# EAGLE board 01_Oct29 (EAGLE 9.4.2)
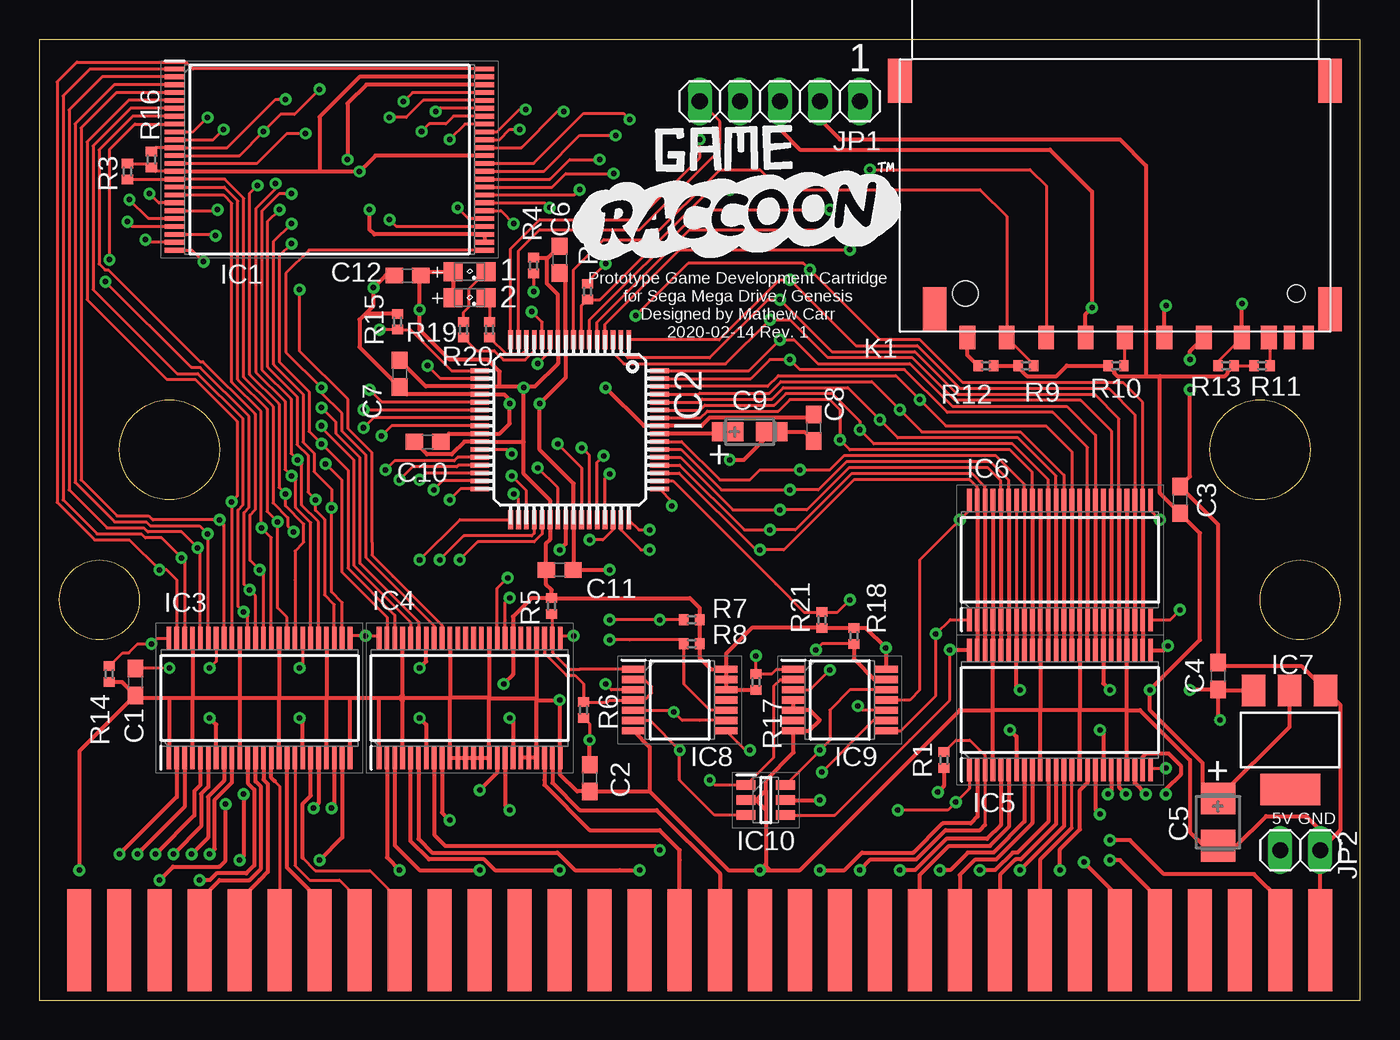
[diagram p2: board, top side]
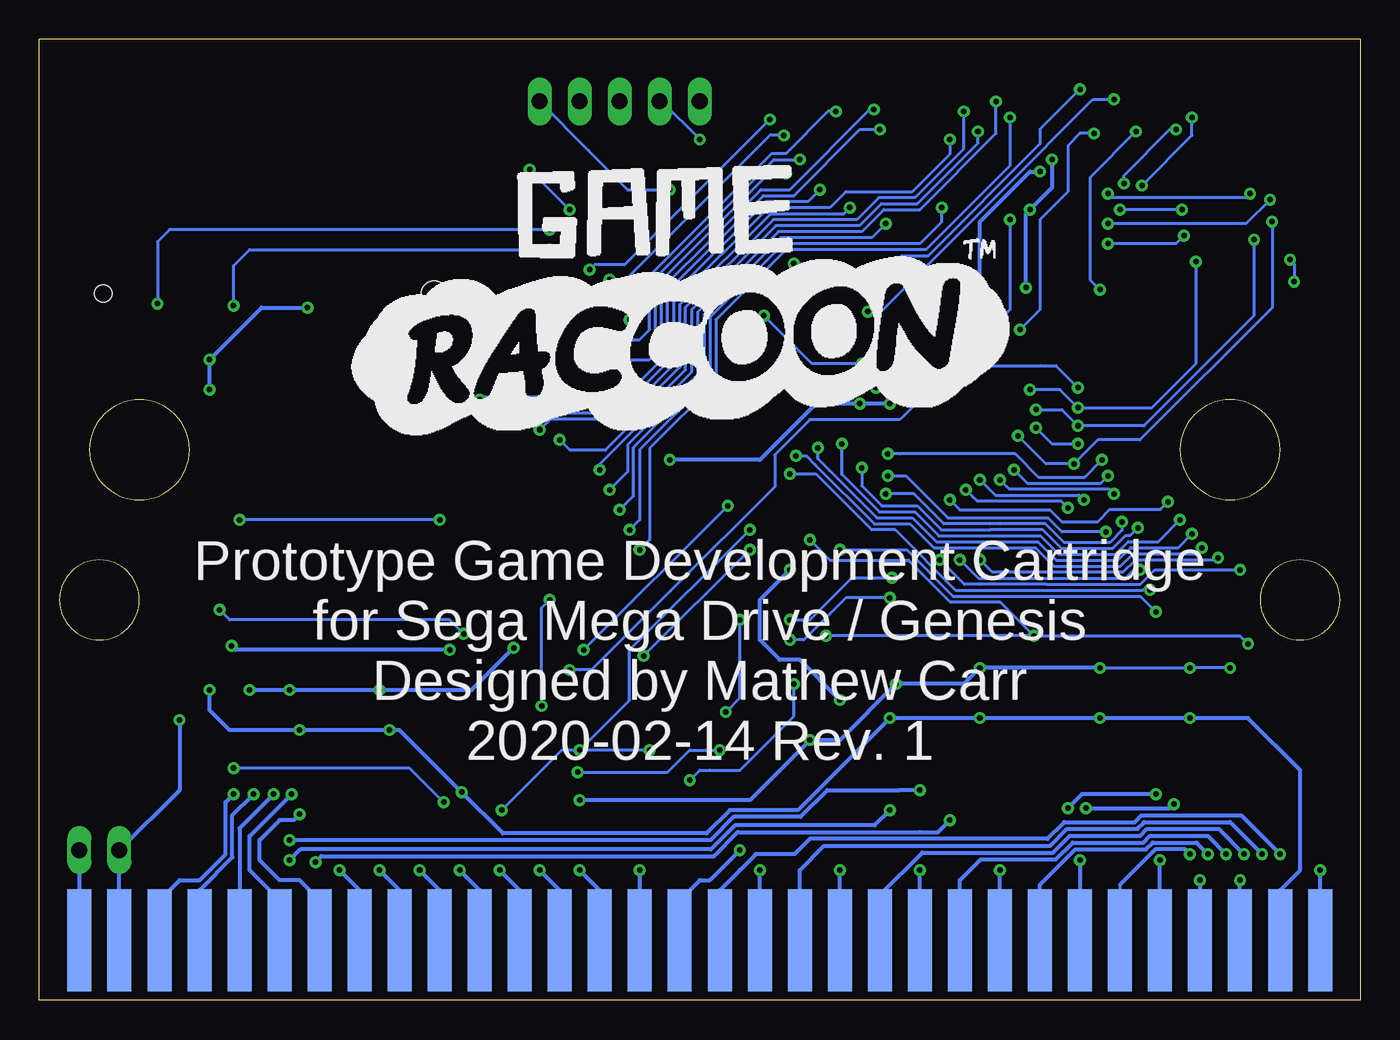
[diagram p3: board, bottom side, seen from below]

Size 83.82 x 60.96 mm. Coordinates in mm from the lower left corner, seen from the top.
Copper layers (1*16): Top 0.035mm / dielectric 1.5mm / Bottom 0.035mm
Design rules "default": minimum track width 6mil, minimum drill 0.35mm, track to track 6mil, track to pad 6mil, pad to pad 6mil, via to via 6mil, smd to smd 6mil, copper to edge 40mil, drill to drill 6mil, minimum pad ring 10mil, minimum via ring 8mil, stop-mask expansion 4mil, vias tented up to drill 0mil, thermal gap 10mil
Net classes: 0 default: width 0.178 mm, clearance 0.178 mm; 1 pow: width 0.254 mm, clearance 0.178 mm

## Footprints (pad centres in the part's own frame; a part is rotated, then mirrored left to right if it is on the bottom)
C0603 = smd 1.1 x 1: 1 -0.85,0; 2 0.85,0
CT3528 = smd 2 x 2.2: + -1.5,0; - 1.5,0
CT3216 = smd 2 x 1.2: + -1.4,0; - 1.4,0
GENESIS-LARGE = smd 1.524 x 6.477 bottom: A1 2.54,3.81; A2 5.08,3.81; A3 7.62,3.81; A4 10.16,3.81; A5 12.7,3.81; A6 15.24,3.81; A7 17.78,3.81; A8 20.32,3.81; A9 22.86,3.81; A10 25.4,3.81; A11 27.94,3.81; A12 30.48,3.81; A13 33.02,3.81; A14 35.56,3.81; A15 38.1,3.81; A16 40.64,3.81; A17 43.18,3.81; A18 45.72,3.81; A19 48.26,3.81; A20 50.8,3.81; A21 53.34,3.81; A22 55.88,3.81; A23 58.42,3.81; A24 60.96,3.81; A25 63.5,3.81; A26 66.04,3.81; A27 68.58,3.81; A28 71.12,3.81; A29 73.66,3.81; A30 76.2,3.81; A31 78.74,3.81; A32 81.28,3.81 | smd 1.524 x 6.477: B1 2.54,3.81; B2 5.08,3.81; B3 7.62,3.81; B4 10.16,3.81; B5 12.7,3.81; B6 15.24,3.81; B7 17.78,3.81; B8 20.32,3.81; B9 22.86,3.81; B10 25.4,3.81; B11 27.94,3.81; B12 30.48,3.81; B13 33.02,3.81; B14 35.56,3.81; B15 38.1,3.81; B16 40.64,3.81; B17 43.18,3.81; B18 45.72,3.81; B19 48.26,3.81; B20 50.8,3.81; B21 53.34,3.81; B22 55.88,3.81; B23 58.42,3.81; B24 60.96,3.81; B25 63.5,3.81; B26 66.04,3.81; B27 68.58,3.81; B28 71.12,3.81; B29 73.66,3.81; B30 76.2,3.81; B31 78.74,3.81; B32 81.28,3.81
SOP50P2000X120-48N = smd 1.25 x 0.3: 1 -9.825,5.75; 2 -9.825,5.25; 3 -9.825,4.75; 4 -9.825,4.25; 5 -9.825,3.75; 6 -9.825,3.25; 7 -9.825,2.75; 8 -9.825,2.25; 9 -9.825,1.75; 10 -9.825,1.25; 11 -9.825,0.75; 12 -9.825,0.25; 13 -9.825,-0.25; 14 -9.825,-0.75; 15 -9.825,-1.25; 16 -9.825,-1.75; 17 -9.825,-2.25; 18 -9.825,-2.75; 19 -9.825,-3.25; 20 -9.825,-3.75; 21 -9.825,-4.25; 22 -9.825,-4.75; 23 -9.825,-5.25; 24 -9.825,-5.75; 25 9.825,-5.75; 26 9.825,-5.25; 27 9.825,-4.75; 28 9.825,-4.25; 29 9.825,-3.75; 30 9.825,-3.25; 31 9.825,-2.75; 32 9.825,-2.25; 33 9.825,-1.75; 34 9.825,-1.25; 35 9.825,-0.75; 36 9.825,-0.25; 37 9.825,0.25; 38 9.825,0.75; 39 9.825,1.25; 40 9.825,1.75; 41 9.825,2.25; 42 9.825,2.75; 43 9.825,3.25; 44 9.825,3.75; 45 9.825,4.25; 46 9.825,4.75; 47 9.825,5.25; 48 9.825,5.75
TQFP64-10X10 = smd 1.2 x 0.3: 1 -5.7,3.75; 2 -5.7,3.25; 3 -5.7,2.75; 4 -5.7,2.25; 5 -5.7,1.75; 6 -5.7,1.25; 7 -5.7,0.75; 8 -5.7,0.25; 9 -5.7,-0.25; 10 -5.7,-0.75; 11 -5.7,-1.25; 12 -5.7,-1.75; 13 -5.7,-2.25; 14 -5.7,-2.75; 15 -5.7,-3.25; 16 -5.7,-3.75; 33 5.7,-3.75; 34 5.7,-3.25; 35 5.7,-2.75; 36 5.7,-2.25; 37 5.7,-1.75; 38 5.7,-1.25; 39 5.7,-0.75; 40 5.7,-0.25; 41 5.7,0.25; 42 5.7,0.75; 43 5.7,1.25; 44 5.7,1.75; 45 5.7,2.25; 46 5.7,2.75; 47 5.7,3.25; 48 5.7,3.75 | smd 0.3 x 1.2: 17 -3.75,-5.7; 18 -3.25,-5.7; 19 -2.75,-5.7; 20 -2.25,-5.7; 21 -1.75,-5.7; 22 -1.25,-5.7; 23 -0.75,-5.7; 24 -0.25,-5.7; 25 0.25,-5.7; 26 0.75,-5.7; 27 1.25,-5.7; 28 1.75,-5.7; 29 2.25,-5.7; 30 2.75,-5.7; 31 3.25,-5.7; 32 3.75,-5.7; 49 3.75,5.7; 50 3.25,5.7; 51 2.75,5.7; 52 2.25,5.7; 53 1.75,5.7; 54 1.25,5.7; 55 0.75,5.7; 56 0.25,5.7; 57 -0.25,5.7; 58 -0.75,5.7; 59 -1.25,5.7; 60 -1.75,5.7; 61 -2.25,5.7; 62 -2.75,5.7; 63 -3.25,5.7; 64 -3.75,5.7
SOP50P810X120-48N = smd 1.475 x 0.3: 1 -3.788,5.75; 2 -3.788,5.25; 3 -3.788,4.75; 4 -3.788,4.25; 5 -3.788,3.75; 6 -3.788,3.25; 7 -3.788,2.75; 8 -3.788,2.25; 9 -3.788,1.75; 10 -3.788,1.25; 11 -3.788,0.75; 12 -3.788,0.25; 13 -3.788,-0.25; 14 -3.788,-0.75; 15 -3.788,-1.25; 16 -3.788,-1.75; 17 -3.788,-2.25; 18 -3.788,-2.75; 19 -3.788,-3.25; 20 -3.788,-3.75; 21 -3.788,-4.25; 22 -3.788,-4.75; 23 -3.788,-5.25; 24 -3.788,-5.75; 25 3.788,-5.75; 26 3.788,-5.25; 27 3.788,-4.75; 28 3.788,-4.25; 29 3.788,-3.75; 30 3.788,-3.25; 31 3.788,-2.75; 32 3.788,-2.25; 33 3.788,-1.75; 34 3.788,-1.25; 35 3.788,-0.75; 36 3.788,-0.25; 37 3.788,0.25; 38 3.788,0.75; 39 3.788,1.25; 40 3.788,1.75; 41 3.788,2.25; 42 3.788,2.75; 43 3.788,3.25; 44 3.788,3.75; 45 3.788,4.25; 46 3.788,4.75; 47 3.788,5.25; 48 3.788,5.75
SOT223 = smd 1.499 x 2.007: 1 -2.261,-3.15; 2 0.025,-3.15; 3 2.311,-3.15 | smd 3.81 x 2.007: 4 0,3.15
SOP65P640X120-14N = smd 1.475 x 0.45: 1 -2.938,1.95; 2 -2.938,1.3; 3 -2.938,0.65; 4 -2.938,0; 5 -2.938,-0.65; 6 -2.938,-1.3; 7 -2.938,-1.95; 8 2.938,-1.95; 9 2.938,-1.3; 10 2.938,-0.65; 11 2.938,0; 12 2.938,0.65; 13 2.938,1.3; 14 2.938,1.95
SOT95P280X145-6N = smd 1.2 x 0.6: 1 -1.25,0.95; 2 -1.25,0; 3 -1.25,-0.95; 4 1.25,-0.95; 5 1.25,0; 6 1.25,0.95
1X05 = drill 1.016 long: 1 -5.08,0; 2 -2.54,0; 3 0,0; 4 2.54,0; 5 5.08,0
1X02 = drill 1.016 long: 1 -1.27,0; 2 1.27,0
693063020911 = smd 1 x 1.5: 1 19.125,0; 2 16.625,0; 3 14.125,0; 4 11.625,0; 5 9.125,0; 6 6.625,0; 7 4.2,0; 8 2.5,0; 9 21.625,0 | smd 0.7 x 1.5: CD 1.2,0; WP 0,0 | smd 1.5 x 2.8: P$12 -1.4,-1.8; P$13 23.7,-1.8; P$14 -1.4,-16.3; P$15 25.9,-16.3 | hole 1.1: 0.75,-2.8 | hole 1.6: 21.75,-2.8
SML0805 = smd 1.2 x 1.2: A 1.05,0; C -1.05,0
R0402 = smd 0.6 x 0.7: 1 -0.5,0; 2 0.5,0

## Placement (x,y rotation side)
C1  100nF  [C0603]  6.1,20.19 270 top
C2  100nF  [C0603]  34.92,14.1 270 top
C3  100nF  [C0603]  72.39,31.75 90 top
C4  100nF  [C0603]  74.8,20.57 270 top
C5  22uF_16V_Tantalum  [CT3528]  74.8,11.3 270 top
C6  100nF  [C0603]  33.02,46.99 270 top
C7  100nF  [C0603]  22.86,39.75 270 top
C8  100nF  [C0603]  49.15,36.32 90 top
C9  10uF_10V_Tantalum  [CT3216]  45.09,36.07 0 top
C10  100nF  [C0603]  24.64,35.43 180 top
C11  100nF  [C0603]  33.02,27.3 0 top
C12  100nF  [C0603]  23.37,45.97 180 top
EDGE1  GENESIS-LARGE  [GENESIS-LARGE]  0,0 0 top
IC1  S29GL064S70TFI030  [SOP50P2000X120-48N]  18.41,53.34 0 top
IC2  PIC24FJ64GA006  [TQFP64-10X10]  33.66,36.2 270 top
IC3  SN74ALVC164245DGGR  [SOP50P810X120-48N]  13.97,19.18 90 top
IC4  SN74ALVC164245DGGR  [SOP50P810X120-48N]  27.3,19.18 90 top
IC5  SN74ALVC164245DGGR  [SOP50P810X120-48N]  64.77,18.41 90 top
IC6  74LVC16374ADGG  [SOP50P810X120-48N]  64.77,27.94 90 top
IC7  REG1117  [SOT223]  79.38,16.51 180 top
IC8  SN74LVC32APW  [SOP65P640X120-14N]  40.64,19.05 0 top
IC9  SN74LVC08APWT  [SOP65P640X120-14N]  50.8,19.05 0 top
IC10  SN74LVC1G11DBVR  [SOT95P280X145-6N]  46.1,12.7 0 top
JP1  [1X05]  46.99,57.02 180 top
JP2  [1X02]  80.01,9.53 0 top
K1  693063020911  [693063020911]  80.52,42.04 180 top
LED1  150080BS75000_BLUE  [SML0805]  27.3,46.23 180 top
LED2  MCL-S270GC_GREEN  [SML0805]  27.3,44.58 180 top
R1  10k  [R0402]  57.4,15.24 90 top
R2  2.2k  [R0402]  34.8,44.96 270 top
R3  10k  [R0402]  5.59,52.58 90 top
R4  10k  [R0402]  31.37,46.61 90 top
R5  10k  [R0402]  32.51,25.02 90 top
R6  10k  [R0402]  34.54,18.41 270 top
R7  10k  [R0402]  41.4,24.13 0 top
R8  10k  [R0402]  41.4,22.61 0 top
R9  10k  [R0402]  62.61,40.26 180 top
R10  10R  [R0402]  68.33,40.26 0 top
R11  10k  [R0402]  77.6,40.26 0 top
R12  10k  [R0402]  60.07,40.26 180 top
R13  10k  [R0402]  75.31,40.26 0 top
R14  10k  [R0402]  4.45,20.7 270 top
R15  10k  [R0402]  22.73,43.05 90 top
R16  10k  [R0402]  7.11,53.34 270 top
R17  10k  [R0402]  45.47,20.19 270 top
R18  10k  [R0402]  51.69,23.11 90 top
R19  330R  [R0402]  26.92,42.55 270 top
R20  150R  [R0402]  28.57,42.55 270 top
R21  10k  [R0402]  49.66,24.13 270 top
U$1  [GAMERACCOONLOGO3_800DPI]  33.15,46.48 0 top
U$2  [GAMERACCOONLOGO2_REVERSEBACK_400DPI]  20.95,34.92 0 top

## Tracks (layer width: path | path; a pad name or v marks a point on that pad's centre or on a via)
CART_!C_CE
  Top 0.203: R5.1 32.55,24.48 IC4.26 32.55,22.05 33.61,21 34.29,21 IC8.1
CART_!C_OE
  Top 0.203: IC8.2 38.41,20.35 38.86,19.9 38.86,19.5 38.41,19.05 IC8.4 36.2,19.05 36.06,18.91 R6.1 34.54,20.07 33.99,20.62 33.45,20.62 32.05,22.02 IC4.27
CART_!LDS  (via drill 0.35)
  Top 0.203: IC8.10 42.56,18.4 40.9,20.06 R8.1 40.65,22.86 37.47,22.86 v36.2,22.86 | IC4.32 29.55,24.13 29.55,25.24 v29.84,25.53
  Bottom 0.203: v29.84,25.53 32.64,25.53 35.31,22.86 v36.2,22.86
CART_!TIME  (via drill 0.35)
  Top 0.203: R7.1 v39.37,24.13 v36.2,24.13 | IC8.9 41.91,17.75 40.8,17.75 v40.26,18.29 40.15,18.4 IC8.5 | IC4.33 29.05,26.13 v29.72,26.8
  Bottom 0.203: v40.26,18.29 39.37,19.18 v39.37,24.13 | v36.2,24.13 34.92,24.13 32.26,26.8 v29.72,26.8
CART_!VRES  (via drill 0.35)
  Top 0.203: R2.1 34.8,45.59 v35.94,46.74 | R4.1 v31.37,44.96 | v17.78,57.78 16.19,56.2 15.3,56.2 v14.22,55.12 12.7,53.59 IC1.12 | v16.51,45.09 16.51,43.18 16.51,41.19 19.58,38.12 19.58,36.27 21.11,34.74 21.11,29.21 21.11,29.06 21.11,28.24 22.45,26.89 25.55,23.79 IC4.40
  Bottom 0.203: v35.94,46.74 33.15,46.74 v31.37,44.96 29.08,47.24 27.4,47.24 20.32,54.33 20.32,55.24 v17.78,57.78 | v14.22,55.12 17.14,52.2 17.14,45.72 v16.51,45.09
CART_A0  (via drill 0.35)
  Top 0.203: IC1.25 17.11,47.59 15.64,46.12 15.64,41.12 v17.91,38.86 17.91,38.52 19.2,37.23 19.2,36.11 20.72,34.58 20.72,28.08 25.05,23.75 IC4.41 | IC2.18 25.45,39.45 v24.64,40.26
  Bottom 0.203: v24.64,40.26 20.32,40.26 19.3,40.26 v17.91,38.86
CART_A1  (via drill 0.35)
  Top 0.203: IC1.24 9.69,47.59 v10.41,46.86 | IC4.43 24.05,24.01 20.34,27.73 20.34,34.42 18.82,35.95 18.82,36.68 v17.91,37.59 | IC2.21 21.75,37.95 v20.95,38.73
  Bottom 0.203: v10.41,46.86 10.41,40.39 13.21,37.59 v17.91,37.59 19.05,38.73 v20.95,38.73
CART_A2  (via drill 0.35)
  Top 0.203: IC1.23 6.9,48.09 v6.73,48.26 | IC4.44 23.55,23.97 19.96,27.57 19.96,34.27 17.91,36.32 v17.91,36.45 | IC2.22 20.59,37.45 v20.57,37.47
  Bottom 0.203: v6.73,48.26 6.73,43.43 13.72,36.45 v17.91,36.45 18.92,37.47 v20.57,37.47
CART_A3  (via drill 0.35)
  Top 0.203: IC1.22 11.1,48.59 v11.18,48.51 | IC4.46 22.55,24.43 19.58,27.41 19.58,33.63 v17.91,35.31 17.12,36.09 17.12,38.62 15.26,40.48 15.26,47.27 v16,48.01 | IC2.23 21.2,36.95 v20.57,36.32
  Bottom 0.203: v11.18,48.51 11.68,48.01 v16,48.01 | v20.57,36.32 19.56,35.31 v17.91,35.31
CART_A4  (via drill 0.35)
  Top 0.203: IC1.21 5.9,49.09 v5.59,49.4 | IC4.47 22.05,24.3 19.2,27.16 19.2,33 v18.16,34.04 | IC2.24 22.35,36.45 v21.72,35.81
  Bottom 0.203: v5.59,49.4 5.59,43.94 13.97,35.56 16.64,35.56 v18.16,34.04 19.94,34.04 v21.72,35.81
CART_A5  (via drill 0.35)
  Top 0.203: IC3.26 19.22,25.23 18.54,25.91 v18.54,31.24 18.54,32.43 17.42,33.55 17.42,34.72 16.74,35.4 16.74,38.46 14.88,40.32 14.88,48.16 v16,49.28 | IC1.20 6.92,49.59 v5.71,50.8 | IC2.31 25.58,32.95 v25.02,32.38
  Bottom 0.203: v5.71,50.8 7.24,49.28 v16,49.28 | v18.54,31.24 18.97,31.67 24.3,31.67 24.57,31.94 v25.02,32.38
CART_A6  (via drill 0.35)
  Top 0.203: IC1.19 11.23,50.09 v11.3,50.16 | v15.24,50.16 14.5,49.43 14.5,40.16 16.36,38.3 16.36,35.24 17.04,34.56 17.04,32.23 v17.53,31.75 17.53,31.08 18.1,30.5 18.1,25.71 18.72,25.09 IC3.27 | IC2.30 24.55,33.45 v24.13,33.02
  Bottom 0.203: v11.3,50.16 v15.24,50.16 | v24.13,33.02 23.16,32.05 17.82,32.05 v17.53,31.75
CART_A7  (via drill 0.35)
  Top 0.203: v16,51.18 15.23,51.18 14.12,50.07 14.12,40 15.98,38.15 15.98,34.7 v16.38,34.29 16.66,34.01 16.66,31.41 17.72,30.35 IC3.29 | IC1.18 7.58,50.59 v6.99,51.18 | IC2.27 29.7,34.95 v29.97,34.67
  Bottom 0.203: v6.99,51.18 7.24,50.93 15.75,50.93 v16,51.18 | v29.97,34.67 29.21,34.67 21.89,34.67 20.4,33.19 17.48,33.19 v16.38,34.29
CART_A8  (via drill 0.35)
  Top 0.203: v4.45,46.99 4.45,53.98 6.06,55.59 IC1.8 | IC3.37 13.72,25.65 v13.34,26.04 12.98,26.39 12.98,30.94 13.31,31.27 13.31,37.04 10.22,40.13 9.65,40.13 v4.19,45.59 | IC2.45 35.91,33.11 v36.2,33.4
  Bottom 0.203: v4.45,46.99 4.19,46.74 v4.19,45.59 | v13.34,26.04 13.77,26.04 13.79,26.01 25.67,26.01 29.5,29.84 30.98,29.84 34.54,33.4 v36.2,33.4
CART_A9  (via drill 0.35)
  Top 0.203: IC3.36 14.22,27.05 v13.97,27.3 13.36,27.91 13.36,30.79 13.69,31.11 13.69,37.2 10.38,40.51 10.2,40.51 4.38,46.33 4.17,46.33 3.79,46.72 3.79,53.95 5.92,56.09 IC1.7 | IC2.36 31.41,29.63 31.24,29.46 26.92,29.46 v25.4,27.94
  Bottom 0.203: v13.97,27.3 14.36,27.3 14.89,26.77 23.5,26.77 24.23,26.77 v25.4,27.94
CART_A10  (via drill 0.35)
  Top 0.203: IC3.38 13.22,24.37 v12.95,24.64 12.6,24.99 12.6,31.1 12.93,31.43 12.93,36.88 10.06,39.75 8.74,39.75 3.4,45.09 3.4,54.2 5.79,56.59 IC1.6
  Top 0.254: v33.02,28.57 33.41,28.96 IC2.40
  Bottom 0.203: v12.95,24.64 13.95,25.63 25.83,25.63 28.77,28.57 v33.02,28.57
CART_A11  (via drill 0.35)
  Top 0.203: IC3.40 12.22,31.59 v12.19,31.62 12.55,31.98 12.55,36.73 9.9,39.37 8.1,39.37 3.02,44.45 3.02,54.46 5.66,57.09 IC1.5 | IC2.32 26.73,32.45 v26.04,31.75
  Bottom 0.203: v12.19,31.62 12.68,31.14 15.88,31.14 16.66,30.35 18.92,30.35 19.68,31.11 25.4,31.11 v26.04,31.75
CART_A12  (via drill 0.35)
  Top 0.203: IC3.41 11.72,30.19 v11.43,30.48 7.19,30.48 6.94,30.73 4.93,30.73 2.64,33.02 2.64,55.35 4.88,57.59 IC1.4 | v32.89,35.31 34.41,33.79 IC2.42
  Bottom 0.203: v11.43,30.48 12.8,29.11 14.72,29.11 15.52,28.3 19.12,28.3 20.29,29.46 26.73,29.46 28.26,30.99 30.51,30.99 32.89,33.37 v32.89,35.31
CART_A13  (via drill 0.35)
  Top 0.203: IC3.43 10.72,29.54 v10.67,29.59 10.16,30.1 7.03,30.1 6.78,30.35 4.77,30.35 2.26,32.86 2.26,55.6 4.75,58.09 IC1.3 | v34.42,35.05 34.91,34.56 IC2.43
  Bottom 0.203: v10.67,29.59 11.53,28.73 14.56,28.73 15.37,27.92 19.28,27.92 20.13,28.77 20.19,28.83 20.44,29.08 24.13,29.08 26.89,29.08 28.41,30.61 30.67,30.61 33.69,33.62 34.42,34.35 v34.42,35.05
CART_A14  (via drill 0.35)
  Top 0.203: IC3.44 10.22,28.52 v10.03,28.7 9.02,29.72 6.88,29.72 6.62,29.97 4.29,29.97 1.88,32.38 1.88,56.49 3.98,58.59 IC1.2 | IC2.44 35.41,34.13 v35.81,34.54
  Bottom 0.203: v10.03,28.7 10.39,28.34 14.4,28.34 15.21,27.54 19.43,27.54 20.6,28.7 23.5,28.7 27.05,28.7 28.57,30.23 30.83,30.23 34.59,33.99 35.14,34.54 v35.81,34.54
CART_A15  (via drill 0.35)
  Top 0.203: IC3.46 9.22,27.86 v9.02,28.07 7.75,29.34 6.72,29.34 6.46,29.59 3.66,29.59 1.5,31.75 1.5,57.38 3.21,59.09 IC1.1 | v24.13,27.94 26.68,30.5 IC2.33
  Bottom 0.203: v9.02,28.07 9.12,27.96 14.24,27.96 15.05,27.16 23.34,27.16 v24.13,27.94
CART_A16  (via drill 0.35)
  Top 0.203: IC3.47 8.72,26.67 8.09,27.3 v7.62,27.3 5.71,29.21 3.5,29.21 1.12,31.59 1.12,58.27 2.37,59.52 9.33,59.52 9.76,59.09 IC1.48 | IC2.37 31.91,29.59 31.4,29.08 27.81,29.08 v26.67,27.94
  Bottom 0.203: v7.62,27.3 13.04,27.3 13.95,26.39 19.68,26.39 19.91,26.39 24.13,26.39 25.12,26.39 v26.67,27.94
CART_A17  (via drill 0.35)
  Top 0.203: IC3.35 14.72,29.35 v14.1,29.97 14.07,30 14.07,37.36 12.21,39.22 12.21,50.56 11.69,51.09 IC1.17 | IC2.39 32.91,32.5 v31.62,33.78
  Bottom 0.203: v14.1,29.97 14.58,29.49 14.87,29.49 15.68,28.68 18.96,28.68 20.13,29.84 23.5,29.84 26.57,29.84 28.1,31.37 30.35,31.37 31.62,32.64 v31.62,33.78
CART_A18  (via drill 0.35)
  Top 0.203: IC1.16 11.73,51.59 12.6,50.72 12.6,39.37 14.45,37.52 14.45,31.01 v15.11,30.35 15.11,27.94 15.11,24.89 15.72,24.29 IC3.33 | IC2.34 30.41,31.82 v30.1,32.13
  Bottom 0.203: v15.11,30.35 15.11,29.8 15.86,29.06 18.8,29.06 19.97,30.23 22.86,30.23 23.5,30.23 26.42,30.23 28.32,32.13 v30.1,32.13
CART_A19  (via drill 0.35)
  Top 0.203: IC1.9 9.75,55.09 v10.67,56.01 | IC3.32 16.22,26.67 16.22,28.5 16.79,29.07 16.79,30.2 15.62,31.37 v15.62,32.13 15.21,32.54 15.21,37.83 13.36,39.69 13.36,51.2 v13.84,51.69 | IC2.29 26.59,33.95 26.49,33.84 23.68,33.84 v22.86,33.02
  Bottom 0.203: v13.84,51.69 10.67,54.86 v10.67,56.01 | v15.62,32.13 15.92,32.43 22.27,32.43 v22.86,33.02
CART_A20  (via drill 0.35)
  Top 0.203: v14.99,51.82 14.99,51.48 13.74,50.23 13.74,39.85 15.6,37.99 15.6,33.68 v16,33.27 16.28,33 16.28,31.25 17.22,30.31 IC3.30 | IC1.10 11.03,54.59 v11.68,55.24 | IC2.28 26.56,34.45 26.33,34.22 22.54,34.22 v21.97,33.66
  Bottom 0.203: v14.99,51.82 14.99,52.32 12.06,55.24 v11.68,55.24 | v21.97,33.66 21.12,32.81 16.47,32.81 v16,33.27
CART_D0  (via drill 0.35)
  Top 0.203: IC2.52 40.64,33.95 44.74,29.84 v46.35,29.84 47.97,29.84 51.53,33.4 59.21,33.4 60.02,32.59 IC6.46 | v26.54,50.29 27.25,49.59 IC1.29
  Top 0.254: IC6.46 IC6.3 IC5.46
  Bottom 0.203: v46.35,29.84 45.72,30.48 45.72,34.92 41.27,39.37 41.27,43.34 36.61,48.01 27.94,48.01 26.54,49.4 v26.54,50.29
CART_D1  (via drill 0.35)
  Top 0.203: IC2.59 41.92,37.45 42.23,37.76 46.65,37.76 47.37,38.48 50.32,38.48 52.07,36.73 v52.07,36.2 52.96,35.31 61.75,35.31 64.02,33.04 IC6.38 | v32.38,50.29 32.09,50.59 IC1.31
  Top 0.254: IC6.38 IC6.11 IC5.38
  Bottom 0.203: v52.07,36.2 51.36,36.91 46.43,36.91 43.18,40.16 43.18,44.13 37.4,49.91 32.77,49.91 v32.38,50.29
CART_D2  (via drill 0.35)
  Top 0.203: IC6.32 67.02,35.85 65.2,37.67 57.96,37.67 55.25,40.39 49.4,40.39 47.88,41.91 v46.99,41.91 45.02,39.95 IC2.64 | v36.45,52.45 33.4,52.45 32.54,51.59 IC1.33
  Top 0.254: IC6.32 IC6.17 IC5.32
  Bottom 0.203: v46.99,41.91 45.72,41.91 45.09,42.55 45.09,44.92 37.55,52.45 v36.45,52.45
CART_D3  (via drill 0.35)
  Top 0.203: IC6.27 69.52,37.16 67.86,38.82 58.43,38.82 55.72,41.53 51.82,41.53 v47.62,45.72 46.96,45.72 43.13,41.9 IC2.1 | v36.58,54.86 34.29,54.86 32.02,52.59 IC1.35
  Top 0.254: IC6.27 IC6.22 IC5.27
  Bottom 0.203: v47.62,45.72 46.61,45.72 37.47,54.86 v36.58,54.86
CART_D4  (via drill 0.35)
  Top 0.203: IC6.29 68.52,36.89 66.97,38.44 58.28,38.44 55.56,41.15 50.29,41.15 v46.99,44.45 46.23,44.45 42.53,40.76 37.35,40.76 36.91,41.2 IC2.2 | v33.27,56.39 32.89,56.39 30.59,54.09 IC1.38
  Top 0.254: IC6.29 IC6.20 IC5.29
  Bottom 0.203: v46.99,44.45 46.63,44.45 37.36,53.72 36.45,53.72 33.78,56.39 v33.27,56.39
CART_D5  (via drill 0.35)
  Top 0.203: IC6.33 66.52,35.08 64.31,37.29 57.62,37.29 54.91,40.01 48.26,40.01 v47.62,40.64 46.35,40.64 45.16,39.45 IC2.63 | v30.86,56.52 30.48,56.52 29.05,55.09 IC1.40
  Top 0.254: IC6.33 IC6.16 IC5.33
  Bottom 0.203: v47.62,40.64 45.09,40.64 44.7,41.02 44.7,44.76 40.6,48.86 38.03,51.44 36.2,51.44 31.11,56.52 v30.86,56.52
CART_D6  (via drill 0.35)
  Top 0.203: IC6.8 IC6.41 62.52,32.73 60.71,34.54 51.05,34.54 50.16,33.66 v48.26,33.66 45.72,33.66 45.09,33.02 43.18,33.02 40.76,35.45 IC2.55 | v24.26,55.12 24.74,55.6 25.8,55.6 26.29,56.09 IC1.42
  Top 0.254: IC6.8 IC5.41
  Bottom 0.203: v48.26,33.66 48.26,34 42.42,39.84 42.42,43.81 37.08,49.15 31.78,49.15 30.38,50.55 28.1,50.55 24.26,54.39 v24.26,55.12
CART_D7  (via drill 0.35)
  Top 0.203: IC2.51 40.6,33.45 45.47,28.57 v45.72,28.57 47.24,28.57 51.69,33.02 59.05,33.02 59.52,32.55 IC6.47 | v22.23,56.01 23.28,56.01 24.36,57.09 IC1.44
  Top 0.254: IC6.47 IC6.2 IC5.47
  Bottom 0.203: v45.72,28.57 45.09,29.21 45.09,30.48 45.09,35.02 40.89,39.21 40.89,43.18 36.45,47.62 27.56,47.62 22.23,52.96 v22.23,56.01
CART_D8  (via drill 0.35)
  Top 0.203: IC2.53 40.68,34.45 44.01,31.11 v46.99,31.11 48.7,31.11 51.37,33.78 60.2,33.78 61.02,32.96 IC6.44 | v30.1,49.28 29.29,50.09 IC1.30
  Top 0.254: IC6.44 IC6.5 IC5.44
  Bottom 0.203: v46.99,31.11 46.1,32 46.1,35.08 41.66,39.53 41.66,43.5 36.77,48.39 30.99,48.39 v30.1,49.28
CART_D9  (via drill 0.35)
  Top 0.203: IC2.61 41.84,38.45 41.92,38.52 46.34,38.52 47.05,39.24 52.83,39.24 v54.61,37.47 56.01,36.07 62.26,36.07 65.02,33.31 IC6.36 | v34.29,51.44 33.95,51.09 IC1.32
  Top 0.254: IC6.36 IC6.13 IC5.36
  Bottom 0.203: v54.61,37.47 54.41,37.67 46.75,37.67 43.94,40.48 43.94,44.44 37.71,50.67 35.05,50.67 v34.29,51.44
CART_D10  (via drill 0.35)
  Top 0.203: IC6.30 68.02,36.12 66.08,38.05 58.12,38.05 55.41,40.77 50.04,40.77 47.62,43.18 v46.35,43.18 43.55,40.37 37.1,40.37 36.41,41.06 IC2.3 | v35.56,53.34 33.66,53.34 32.41,52.09 IC1.34
  Top 0.254: IC6.30 IC6.19 IC5.30
  Bottom 0.203: v46.35,43.18 45.47,44.07 45.47,45.07 37.2,53.34 v35.56,53.34
CART_D11  (via drill 0.35)
  Top 0.203: IC6.26 70.02,37.93 68.75,39.2 58.59,39.2 55.88,41.91 53.34,41.91 v48.9,46.35 48.49,46.76 41.17,46.76 v37.85,43.43 | IC2.11 32.41,41.17 v31.62,40.39 | v37.47,55.88 37.08,56.26 34.54,56.26 31.37,53.09 IC1.36
  Top 0.254: IC6.26 IC6.23 IC5.26
  Bottom 0.203: v31.62,40.39 34.8,40.39 v37.85,43.43 | v48.9,46.35 48.6,46.65 46.7,46.65 v37.47,55.88
CART_D12  (via drill 0.35)
  Top 0.203: IC6.35 65.52,34.81 63.88,36.45 57.53,36.45 v55.88,38.1 54.36,39.62 46.9,39.62 46.22,38.95 IC2.62 | v30.48,55.24 29.84,55.24 29.19,54.59 IC1.39
  Top 0.254: IC6.35 IC6.14 IC5.35
  Bottom 0.203: v55.88,38.1 55.69,38.29 46.67,38.29 44.32,40.63 44.32,44.6 37.87,51.05 35.94,51.05 31.75,55.24 v30.48,55.24
CART_D13  (via drill 0.35)
  Top 0.203: IC2.60 41.88,37.95 42.08,38.14 46.49,38.14 47.21,38.86 51.31,38.86 v53.34,36.83 54.48,35.69 62.1,35.69 64.52,33.27 IC6.37 | v26.04,54.61 27.02,55.59 IC1.41
  Top 0.254: IC6.37 IC6.12 IC5.37
  Bottom 0.203: v53.34,36.83 52.88,37.29 46.59,37.29 43.56,40.32 43.56,44.28 37.55,50.29 33.66,50.29 32.64,51.31 28.41,51.31 26.04,53.69 v26.04,54.61
CART_D14  (via drill 0.35)
  Top 0.203: IC2.58 41.96,36.95 42.39,37.38 46.9,37.38 47.62,38.1 50.16,38.1 50.8,37.47 v50.8,35.56 51.44,34.92 61.59,34.92 63.02,33.5 IC6.40 | IC1.43 25.35,56.59 v25.15,56.39
  Top 0.254: IC6.40 IC6.9 IC5.40
  Bottom 0.203: v25.15,56.39 25.15,54.04 28.26,50.93 30.54,50.93 31.94,49.53 37.24,49.53 42.8,43.97 42.8,40 47.88,34.92 50.16,34.92 v50.8,35.56
CART_D15  (via drill 0.35)
  Top 0.203: IC2.54 40.72,34.95 43.28,32.38 v47.62,32.38 49.43,32.38 51.21,34.16 60.36,34.16 61.52,33 IC6.43 | v23.11,57.02 23.68,57.59 IC1.45
  Top 0.254: IC6.43 IC6.6 IC5.43
  Bottom 0.203: v47.62,32.38 46.48,33.53 46.48,35.24 42.04,39.69 42.04,43.65 36.92,48.77 31.62,48.77 30.23,50.16 27.94,50.16 23.11,54.99 v23.11,57.02
DATATRANSCEIVER!OE  (via drill 0.35)
  Top 0.203: IC10.4 50.48,11.75 55.24,16.51 57.78,19.05 v57.78,22.23
  Top 0.254: IC5.25 71.35,22.2 v71.63,22.48 | v57.78,22.23 59,22.23 IC5.48
  Bottom 0.254: v57.78,22.23 71.37,22.23 v71.63,22.48
EDGE_!C_CE
  Top 0.254: EDGE1.B17 43.18,8.05 39.17,12.06 34.29,12.06 32.55,13.8 IC4.23
EDGE_!C_OE
  Top 0.254: EDGE1.B16 40.64,8.89 40.64,9.53 39.37,10.79 34.92,10.79 32.05,13.66 32.05,13.97 IC4.22
EDGE_!LDS  (via drill 0.35)
  Top 0.254: EDGE1.B28 71.12,6.35 68.58,8.89 v67.94,8.89 | IC4.17 29.55,12.36 v29.84,12.06
  Bottom 0.254: v67.94,8.89 67.26,9.58 41.2,9.58 39.68,11.1 30.81,11.1 v29.84,12.06
EDGE_!TIME  (via drill 0.35)
  Top 0.254: EDGE1.B31 78.74,6.35 77.09,8 71.37,8 69.22,10.16 v67.94,10.16 | IC4.16 29.05,14.45 v27.94,13.34
  Bottom 0.254: v67.94,10.16 41.23,10.16 39.75,11.63 35.51,11.63 33.81,13.34 29.21,13.34 v27.94,13.34
EDGE_!VRES  (via drill 0.35)
  Top 0.254: EDGE1.B27 68.58,6.48 v66.29,8.76 | IC4.9 25.55,11.91 v26.04,11.43
  Bottom 0.254: v66.29,8.76 65.91,9.14 41.02,9.14 39.5,10.66 27.94,10.66 26.8,10.66 v26.04,11.43
EDGE_A1  (via drill 0.35)
  Top 0.254: IC4.8 25.05,10.51 25.76,9.8 39.09,9.8 v39.37,9.53
  Bottom 0.254: v39.37,9.53 41.27,7.62 41.91,7.62 43.18,6.35 EDGE1.A17
EDGE_A2  (via drill 0.35)
  Top 0.254: v38.1,8.26 36.83,8.26 33.99,8.26 32.87,9.37 24.92,9.37 24.05,10.23 IC4.6
  Bottom 0.254: EDGE1.A15 v38.1,8.26
EDGE_A3  (via drill 0.35)
  Top 0.254: v33.02,8.26 28.91,8.26 28.22,8.94 24.72,8.94 23.55,10.1 IC4.5
  Bottom 0.254: EDGE1.A13 v33.02,8.26
EDGE_A4  (via drill 0.35)
  Top 0.254: v27.94,8.26 24.13,8.26 22.55,9.83 IC4.3
  Bottom 0.254: EDGE1.A11 v27.94,8.26
EDGE_A5  (via drill 0.35)
  Top 0.254: v22.86,8.26 22.05,9.06 IC4.2
  Bottom 0.254: EDGE1.A9 v22.86,8.26
EDGE_A6  (via drill 0.35)
  Top 0.254: IC3.23 19.22,12.48 19.23,12.47 19.23,10.34 v17.78,8.89
  Bottom 0.254: v17.78,8.89 EDGE1.A7
EDGE_A7  (via drill 0.35)
  Top 0.254: v12.95,13.08 12.95,9.14 v12.7,8.89 | IC3.22 18.72,12.37 v18.54,12.19
  Bottom 0.254: EDGE1.A5 v12.7,8.89 | v12.95,13.08 17.65,13.08 v18.54,12.19
EDGE_A8  (via drill 0.35)
  Top 0.254: v7.62,7.62 8.48,8.48 11.43,8.48 11.81,8.87 v11.81,12.45 | IC3.20 17.72,12.51 v17.4,12.19
  Bottom 0.254: EDGE1.A3 v7.62,7.62 | v17.4,12.19 12.06,12.19 v11.81,12.45
EDGE_A9
  Top 0.254: EDGE1.B4 10.16,6.35 11.43,7.62 13.34,7.62 14.07,8.35 14.07,13.54 13.81,13.81 13.72,13.89 IC3.12
EDGE_A10
  Top 0.254: EDGE1.B5 12.7,6.35 13.97,7.62 14.5,8.15 14.5,13.72 14.22,14 IC3.13
EDGE_A11  (via drill 0.35)
  Top 0.254: v10.16,7.62 10.82,7.62 11.25,8.05 13.13,8.05 13.64,8.56 13.64,13.36 13.22,13.78 IC3.11
  Bottom 0.254: v10.16,7.62 EDGE1.A4
EDGE_A12  (via drill 0.35)
  Top 0.254: v10.79,9.27 11.13,9.6 11.13,12.73 12.22,13.82 IC3.9
  Bottom 0.203: 15.24,7.32 EDGE1.A6
  Bottom 0.254: v10.79,9.27 11.1,9.57 12.98,9.57 15.24,7.32
EDGE_A13  (via drill 0.35)
  Top 0.254: IC3.8 11.72,13.93 10.7,12.91 10.7,10.31 v9.65,9.27
  Bottom 0.254: EDGE1.A8 20.32,7.32 18.06,9.57 13.59,9.57 13.16,10.01 10.39,10.01 v9.65,9.27
EDGE_A14  (via drill 0.35)
  Top 0.254: IC3.6 10.72,13.54 10.26,13.09 10.26,11.03 v8.51,9.27
  Bottom 0.254: EDGE1.A10 25.4,7.62 24.08,8.94 19.31,8.94 18.24,10.01 13.77,10.01 13.34,10.44 9.68,10.44 v8.51,9.27
EDGE_A15  (via drill 0.35)
  Top 0.254: IC3.5 10.22,13.65 9.83,13.27 9.83,11.74 v7.37,9.27
  Bottom 0.254: EDGE1.A12 30.48,6.68 27.79,9.37 19.49,9.37 18.42,10.44 13.95,10.44 13.52,10.87 8.96,10.87 v7.37,9.27
EDGE_A16  (via drill 0.35)
  Top 0.254: IC3.3 9.22,12.27 v6.22,9.27
  Bottom 0.254: EDGE1.A14 35.56,8.26 34.01,9.8 19.67,9.8 18.6,10.87 14.13,10.87 13.7,11.3 8.25,11.3 v6.22,9.27
EDGE_A17  (via drill 0.35)
  Top 0.254: IC3.2 8.72,12.91 v5.08,9.27
  Bottom 0.254: v5.08,9.27 7.54,11.73 13.88,11.73 14.31,11.3 18.78,11.3 19.84,10.23 34.92,10.23 35.89,9.27 38.35,9.27 39.37,8.26 40.64,6.99 EDGE1.A16
EDGE_A18
  Top 0.203: 14.93,13.9 15.24,13.59 EDGE1.B6
  Top 0.254: 14.93,13.9 14.72,14.11 IC3.14
EDGE_A19
  Top 0.254: EDGE1.B7 17.78,6.35 15.72,8.41 IC3.16
EDGE_A20
  Top 0.203: IC3.17 16.22,8.54 17.14,7.62 19.05,7.62 20.32,6.35
  Top 0.254: EDGE1.B8 20.32,4.45 20.32,6.35
EDGE_A21
  Top 0.203: 16.73,9.01 17.51,8.23 20.98,8.23 22.86,6.35
  Top 0.254: 22.86,6.35 EDGE1.B9 | IC3.19 17.22,12.98 16.72,12.47 16.72,9.02 16.73,9.01
EDGE_D0  (via drill 0.35)
  Top 0.203: R1.2 58.17,16.51 58.42,16.51 59.05,16.51 60.02,15.54 IC5.3 60.02,11.12
  Top 0.254: v52.07,8.26 52.75,8.94 55.65,8.94 57.5,10.79 59.69,10.79 60.02,11.12
  Bottom 0.254: EDGE1.A20 50.8,6.99 v52.07,8.26
EDGE_D1  (via drill 0.35)
  Top 0.254: v59.69,8.26 60.65,8.26 61.77,9.37 62.08,9.37 64.02,11.31 IC5.11
  Bottom 0.254: EDGE1.A23 58.42,6.99 v59.69,8.26
EDGE_D2  (via drill 0.35)
  Top 0.254: IC5.17 67.02,12.1 v67.31,11.81
  Bottom 0.254: v67.31,11.81 67.69,11.43 68.58,11.43 69.85,10.16 69.85,8.89 68.58,7.62 67.31,7.62 66.04,6.35 EDGE1.A26
EDGE_D3  (via drill 0.35)
  Top 0.254: IC5.22 69.52,13.79 v70.23,13.08
  Bottom 0.254: EDGE1.A29 73.66,6.99 71.57,9.07 71.57,11.74 v70.23,13.08
EDGE_D4  (via drill 0.35)
  Top 0.254: IC5.20 68.52,13.52 v68.96,13.08
  Bottom 0.254: v68.96,13.08 71.12,10.92 EDGE1.A28
EDGE_D5  (via drill 0.35)
  Top 0.254: v64.77,8.26 64.77,9.57 66.04,10.84 66.04,13.34 66.29,13.59 66.3,13.59 66.52,13.81 IC5.16
  Bottom 0.254: EDGE1.A25 63.5,6.99 v64.77,8.26
EDGE_D6  (via drill 0.35)
  Top 0.254: v57.15,8.26 57.81,8.26 58.92,9.37 60.55,9.37 62.52,11.34 IC5.8
  Bottom 0.254: EDGE1.A22 55.88,6.99 v57.15,8.26
EDGE_D7  (via drill 0.35)
  Top 0.254: IC5.2 59.54,14.6 59.54,11.66 59.11,11.23 57.32,11.23 55.47,9.37 52.22,9.37 51.1,8.26 v49.53,8.26
  Bottom 0.254: EDGE1.A19 48.26,6.99 v49.53,8.26
EDGE_D8  (via drill 0.35)
  Top 0.254: v54.61,8.26 55.57,8.26 57.55,10.23 60.15,10.23 61.02,11.11 IC5.5
  Bottom 0.254: EDGE1.A21 53.34,6.99 v54.61,8.26
EDGE_D9  (via drill 0.35)
  Top 0.254: v62.23,8.26 65.02,11.04 IC5.13
  Bottom 0.254: EDGE1.A24 60.96,6.99 v62.23,8.26
EDGE_D10  (via drill 0.35)
  Top 0.254: IC5.19 68.02,13.28 v67.82,13.08
  Bottom 0.254: EDGE1.A27 68.58,6.35 70.48,8.26 70.48,10.41 v67.82,13.08
EDGE_D11  (via drill 0.35)
  Top 0.254: v71.5,13.08 71.5,13.38 72.44,14.32 72.44,14.89 71.66,15.67 70.24,15.67 70.02,15.45 IC5.23
  Bottom 0.254: EDGE1.A30 76.2,6.35 74.93,7.62 73.66,7.62 72.01,9.27 72.01,12.58 v71.5,13.08
EDGE_D12
  Top 0.203: 65.52,10.93 IC5.14
  Top 0.254: EDGE1.B25 63.5,8.91 65.39,10.81 65.52,10.93
EDGE_D13
  Top 0.254: EDGE1.B24 60.96,7.95 61.95,8.94 62.28,8.94 64.52,11.18 IC5.12
EDGE_D14
  Top 0.254: EDGE1.B23 58.42,7.95 59.41,8.94 60.73,8.94 63.02,11.23 IC5.9
EDGE_D15
  Top 0.254: EDGE1.B22 55.88,7.95 57.73,9.8 60.33,9.8 61.52,11 IC5.6
FLASH_!EXTERNALOE  (via drill 0.35)
  Top 0.203: IC8.3 36.31,19.7 v35.94,20.07 | IC9.2 47.02,20.35 46.61,19.94 46.61,15.41 IC10.1 42.87,13.65 v42.55,13.97
  Bottom 0.203: v42.55,13.97 41.91,14.61 41.27,14.61 39.37,14.61 35.94,18.03 v35.94,20.07
FLASH_!OE  (via drill 0.35)
  Top 0.203: v22.23,49.53 22.66,49.09 IC1.28 | IC9.3 48.91,19.7 v50.16,20.95
  Bottom 0.203: v22.23,49.53 22.23,43.81 29.21,36.83 33.66,36.83 34.92,36.83 37.15,34.61 37.15,32.58 43.75,25.97 48.77,20.95 49.53,20.95 v50.16,20.95
GND  (via drill 0.35)
  Top 0.254: IC3.45 9.72,19.18 | IC3.4 9.72,19.18 | IC3.39 12.72,19.18 | 12.72,19.18 IC3.10 | IC3.34 15.22,19.18 | IC3.15 15.22,19.18 | IC3.28 18.22,19.18 | IC3.21 18.22,19.18 | 8.26,19.18 9.72,19.18 | 9.72,19.18 12.72,19.18 | 12.72,19.18 15.22,19.18 | 15.22,19.18 18.22,19.18 | IC3.1 8.26,15.42 8.26,19.18 | 18.22,19.18 19.68,19.18 | 19.68,19.18 21.59,19.18 | 21.59,19.18 22.86,19.18 | IC3.24 19.72,19.14 19.68,19.18 | IC4.1 21.55,19.14 21.59,19.18 | 22.86,19.18 23.05,19.37 IC4.45 | IC4.4 23.05,18.98 22.86,19.18 | 22.86,19.18 26.04,19.18 | 28.57,19.18 26.04,19.18 | IC4.39 26.05,19.2 26.04,19.18 | IC4.34 28.55,19.2 28.57,19.18 | EDGE1.B32 JP2.2 | IC5.4 60.52,18.41 | 60.52,18.41 IC5.45 IC6.4 IC6.45 | IC6.39 IC6.10 IC5.39 63.52,18.41 | IC6.34 IC6.15 IC5.34 66.02,18.41 | IC6.28 IC6.21 IC5.28 69.02,18.41 | IC5.15 66.02,18.41 | IC5.10 63.52,18.41 | 69.02,18.41 66.02,18.41 | 66.02,18.41 63.52,18.41 | 63.52,18.41 60.52,18.41 | 69.02,18.41 69.85,18.41 73.03,15.24 73.03,10.67 73.89,9.8 C5.- 75.97,9.8 77.85,11.68 80.39,11.68 81.28,10.79 JP2.2 | C1.2 2.54,15.79 v2.54,8.26 | C1.2 6.26,19.18 8.26,19.18 | v73.03,40.64 73.03,41.17 K1.6 | v73.03,38.73 73.03,33.23 C3.2 74.8,30.19 C4.1 75.02,21.21 80.09,21.21 IC7.1 82.55,18.75 82.55,10.79 JP2.2 | R14.2 5.24,20.2 C1.2 | 33.91,27.34 IC2.41 33.91,32.77 31.75,34.92 v31.75,37.85 33.41,39.5 IC2.9 33.41,45.76 C6.2 | 33.91,27.34 C11.2 | C10.1 26,35.95 IC2.25 29.21,35.95 29.84,36.58 v29.84,37.85 29.84,38.1 29.5,38.45 IC2.20 23.32,38.45 C7.2 20.32,41.44 20.32,43.18 20.69,43.55 | v19.56,53.34 19.56,56.9 20.75,58.09 IC1.46 | v43.81,34.29 44.71,34.29 C9.- 48.55,36.07 C8.1 | K1.3 66.39,43.53 v66.8,43.94 66.8,51.31 64.14,53.98 48.26,53.98 46.99,55.24 JP1.3
  Top 0.254: IC5.21 69.02,18.41 | R15.2 20.69,43.55 | 20.69,43.55 21.21,44.07 v21.21,45.21 21.97,45.97 C12.2 | IC1.26 IC1.27 21.26,48.59 20.95,48.9 v20.95,50.16 | 26.04,19.18 26.05,19.16 IC4.10 IC4.11 IC4.12 IC4.13 IC4.14 IC4.15 28.55,19.16 | 28.57,19.18 28.55,19.16 | v45.72,8.26 43.73,8.26 38.73,13.25 | 38.73,13.25 C2.2 34.12,13.25 33.05,14.32 IC4.24 33.05,19.02 v33.02,19.05 31.55,19.05 | IC9.4 IC9.5 48.91,18.4 49.53,17.78 48.85,17.1 IC9.7 47.86,15.73 46.1,13.97 46.1,13.34 | 45.47,12.7 46.1,13.34 | IC8.7 38.73,16.07 38.73,13.25 | 46.1,13.34 46.1,12.06 | 46.1,12.06 46.1,8.64 | v45.72,8.26 46.1,8.64 | IC10.2 45.47,12.7 | 45.47,12.7 46.1,12.06 | IC4.28 31.55,19.05 | 31.55,19.05 IC4.21 IC4.20 IC4.19 | 28.55,19.16 31.45,19.16 31.55,19.05 | 33.91,27.34 33.94,27.3 v36.2,27.3 | v45.72,8.26 46.35,8.26 | 46.35,8.26 48.26,8.26 58.42,18.41 60.52,18.41 | 46.1,8.64 46.1,8.51 46.35,8.26
  Bottom 0.254: EDGE1.A1 v2.54,8.26 | JP2.2 EDGE1.B32 | v73.03,38.73 v73.03,40.64 69.72,43.94 v66.8,43.94 | v19.56,53.34 19.56,51.56 v20.95,50.16 21.21,49.91 v21.21,45.21 | v43.81,34.29 38.1,34.29 34.54,37.85 v31.75,37.85 v29.84,37.85 | v45.72,8.26 EDGE1.A18 | v33.02,19.05 35.56,21.59 36.83,21.59 38.1,22.86 38.1,25.4 v36.2,27.3
MCU_!68000  (via drill 0.35)
  Top 0.203: R14.1 5.29,22.05 5.68,22.05 6.24,22.61 v7.11,22.61 7.47,22.96 IC3.48 | IC3.25 19.87,23.11 v20.7,23.11 21.41,23.11 IC4.48 | IC4.25 33.2,23.11 v33.91,23.11 | IC2.46 36.41,29.85 35.77,29.21 v34.92,29.21
  Bottom 0.203: v20.7,23.11 7.62,23.11 v7.11,22.61 | v20.7,23.11 v33.91,23.11 | v20.7,23.11 22.84,25.25 25.99,25.25 27.36,26.62 28.66,27.92 33.63,27.92 v34.92,29.21
MCU_!LEDBLUE
  Top 0.203: IC2.13 31.41,41.21 30.83,40.63 29.45,40.63 28.87,41.21 27.76,41.21 R19.2
MCU_!LEDGREEN
  Top 0.203: IC2.14 30.91,41.25 30.67,41.02 29.6,41.02 R20.2
MCU_!MCLR  (via drill 0.35)
  Top 0.203: IC2.7 34.41,44.06 R2.2 35.57,44.46 42.55,51.44 v43.81,51.44
  Bottom 0.203: JP1.1 48.96,53.91 46.48,51.44 v43.81,51.44
MCU_FLASH!OE  (via drill 0.35)
  Top 0.203: v45.47,21.84 R17.1 46.47,20.69 46.74,20.95 47.82,20.95 IC9.1 | IC2.47 36.91,29.85 38.18,28.57 v38.73,28.57
  Bottom 0.203: v45.47,21.84 v38.73,28.57
MCU_FLASH!WE  (via drill 0.35)
  Top 0.203: R16.1 7.36,54.09 IC1.11 11.93,54.09 14.99,57.15 v15.62,57.15 | IC2.12 31.91,43.02 v31.24,43.69
  Bottom 0.203: v31.24,43.69 30.42,43.69 22.77,51.34 16.96,57.15 16.51,57.15 v15.62,57.15
MCU_FLASHREADY  (via drill 0.35)
  Top 0.203: v16.13,29.72 15.77,30.08 15.77,30.62 14.83,31.56 14.83,37.67 12.98,39.53 12.98,50.88 11.77,52.09 IC1.15 8.58,52.08 R3.1 | IC2.35 30.91,32.34 v29.97,33.27
  Bottom 0.203: v16.13,29.72 18.92,29.72 19.81,30.61 24.13,30.61 26.16,30.61 28.83,33.27 v29.97,33.27
MCU_GAME/!BOOT  (via drill 0.35)
  Top 0.203: IC1.13 13.82,53.09 15.72,54.99 v16.89,54.99 | v21.59,42.55 v21.6,42.55 R15.1 23.55,42.55 26.16,39.95 IC2.17
  Bottom 0.203: v16.89,54.99 17.78,54.99 18.54,54.23 18.54,51.31 19.68,50.16 20.32,49.53 20.32,43.81 v21.59,42.55
MCU_REGISTER!INTERNALOE  (via drill 0.35)
  Top 0.203: IC2.50 40.21,32.95 46.74,26.42 48.52,24.63 R21.1 50.66,24.63 v51.44,25.4 | IC9.10 52.21,18.4 v51.94,18.67
  Bottom 0.203: v51.94,18.67 51.94,24.89 v51.44,25.4
MCU_REGISTERINTERNALCLK  (via drill 0.35)
  Top 0.203: R18.1 49.66,22.61 v49.28,22.23 | IC2.49 40.13,31.67 v40.13,31.37
  Top 0.254: IC9.13 52.99,20.35 51.69,21.66 R18.1
  Bottom 0.203: v49.28,22.23 v40.13,31.37
MCU_VCAP_TANTALUM
  Top 0.254: C9.+ 43.56,35.95 IC2.56
N$4
  Top 0.203: LED1.C 27.26,45.13 27.26,43.99 26.92,43.65 R19.1
N$5
  Top 0.203: LED2.C 28.57,44.36 R20.1
PICKITCLOCK
  Top 0.203: JP1.5 43.18,55.75 43.18,53.98 38.1,48.9 31.75,48.9 30.41,47.55 IC2.15
PICKITDATA  (via drill 0.35)
  Top 0.203: v41.91,54.61 41.91,53.47 37.97,49.53 31.75,49.53 29.91,47.69 IC2.16
  Bottom 0.203: v41.91,54.61 44.32,57.02 JP1.4
REGISTER_!EXTERNALOE  (via drill 0.35)
  Top 0.203: IC10.3 42.86,11.75 40.64,13.97 v40.64,15.88 38.77,17.75 IC8.6 | IC9.9 52.93,17.75 v49.66,14.48
  Bottom 0.203: v40.64,15.88 42.55,15.88 43.94,14.48 v49.66,14.48
REGISTER_!OE  (via drill 0.35)
  Top 0.203: IC6.24 71.78,24.15 v72.39,24.77 | IC9.8 54.69,17.1 56.9,19.3 v56.9,23.24 57.81,24.15 IC6.1
  Bottom 0.203: v56.9,23.24 57.78,24.13 71.75,24.13 v72.39,24.77
REGISTERCLK  (via drill 0.35)
  Top 0.203: IC6.25 70.52,31.08 v71.12,30.48 | IC6.48 59.02,31.08 v58.42,30.48 57.15,29.21 55.88,27.94 55.88,19.68 55.24,19.05 IC9.11
  Bottom 0.203: v58.42,30.48 v71.12,30.48
REGISTEREXTERNALCLK  (via drill 0.35)
  Top 0.203: IC9.12 53.72,19.68 51.44,19.68 50.16,18.41 50.16,16.51 v49.53,15.88 49.53,15.83 IC10.6 | IC8.8 44.8,15.88 v45.09,15.88 | IC5.1 59.02,13.43 v58.17,12.57 57.66,12.06 v54.48,12.06 | IC2.48 38.05,29.84 v38.73,29.84 | IC5.24 70.62,14.73 v71.5,14.73
  Bottom 0.203: v45.09,15.88 v49.53,15.88 | v49.53,15.88 50.67,15.88 v54.48,12.06 | v49.53,15.88 46.35,19.05 46.35,22.23 v38.73,29.84 | v71.5,14.73 60.33,14.73 v58.17,12.57
SD4_VCC3V3_10R
  Top 0.203: R10.2 68.89,40.33 K1.4
SD8_PULLUP
  Top 0.203: K1.8 78.1,41.96 R11.2
SD9_PULLUP
  Top 0.254: R12.2 58.89,40.94 K1.9
SPI2!SS
  Top 0.203: IC2.8 33.91,46.35 35.81,48.26 38.73,48.26 43.18,52.7 45.72,52.7 46.99,51.44 59.69,51.44 61.39,49.73 K1.1 63.11,40.32 R9.1
SPI2CLK  (via drill 0.35)
  Top 0.203: IC2.4 35.91,42.89 40.64,47.62 v51.44,47.62
  Top 0.254: K1.5 71.39,43.96 v71.5,44.07
  Bottom 0.203: v71.5,44.07 71.5,46.61 70.48,47.62 v51.44,47.62
SPI2MISO  (via drill 0.35)
  Top 0.203: R13.1 74.81,40.53 K1.7 | IC2.5 35.41,43.02 41.27,48.9 46.99,48.9 v51.44,48.9
  Top 0.254: K1.7 76.32,44.19 v76.33,44.2
  Bottom 0.203: v51.44,48.9 75.56,48.9 76.33,48.13 v76.33,44.2
SPI2MOSI  (via drill 0.35)
  Top 0.203: IC2.6 34.91,43.16 41.91,50.16 v50.16,50.16 | v52.7,52.7 62.87,52.7 63.89,51.68 K1.2
  Bottom 0.203: v50.16,50.16 v52.7,52.7
VCC3V3  (via drill 0.35)
  Top 0.203: IC3.42 11.22,21.51 v10.79,21.08 | IC3.31 16.72,21.29 v16.51,21.08 | C1.1 6.13,21.08 v8.26,21.08 | R13.2 R11.1 | IC6.42 IC6.7 | IC1.14 7.36,52.59 R16.2 6.87,53.08 R3.2 | R6.2 34.92,17.53 v34.92,16.51
  Top 0.254: v24.13,21.08 24.55,21.51 IC4.42 | IC6.31 IC6.18 IC5.31 67.52,20.11 v67.94,19.68 | IC6.7 IC5.42 62.02,19.89 v62.23,19.68 | IC7.2 79.35,17.35 C5.+ 73.83,13.78 73.83,15.05 70.48,18.39 v70.48,19.68 73.66,22.86 73.66,29.63 C3.1 71.12,32.17 71.12,39.6 | R13.2 75.42,39.86 75.42,39.78 75.24,39.6 71.12,39.6 | 70.23,39.6 68.4,39.6 68.22,39.78 68.22,39.86 R10.1 65.21,40.26 64.55,39.6 62.69,39.6 62.11,40.18 R9.2 R12.1 | 70.23,39.6 71.12,39.6 | C8.2 48.95,36.97 42.56,36.97 42.03,36.45 IC2.57 38.36,36.45 v35.94,38.86 | C7.1 24.52,38.95 IC2.19 29.21,38.95 | C10.2 24.59,34.63 26.16,34.63 26.98,35.45 IC2.26 30.72,35.45 30.73,35.43 | 29.21,38.95 29.21,39.88 28.45,40.64 26.04,40.64 24.13,42.55 v24.13,43.81 24.13,45.89 C12.1 24.47,46.23 LED1.A LED2.A | IC1.14 17.78,52.59 | 32.28,47.1 32.22,47.03 32.22,45.46 32.91,44.77 IC2.10 32.91,40.4 31.43,38.92 30.67,38.92 | 32.28,47.1 C6.1 | R4.2 32.27,47.11 32.28,47.1 | 29.21,38.95 30.65,38.95 30.67,38.92 | 30.67,38.92 v30.73,38.86 30.73,35.43 | 30.73,35.43 30.73,33.4 32.41,31.73 IC2.38 32.41,29.23 32.13,28.96 32.13,27.34 C11.1 32.17,26.38 32.51,26.04 R5.2 | IC1.47 20.32,58.59 17.78,56.05 17.78,52.59 | 17.78,52.59 20.31,52.59 v20.32,52.58 21.33,53.59 IC1.37 | JP1.2 49.53,55.88 50.8,54.61 68.58,54.61 70.23,52.96 70.23,39.6 | v29.46,20.07 30.05,20.66 IC4.31 30.05,24.34 31.23,25.52 R5.2 | C2.1 v34.92,16.51 | IC10.5 v49.53,12.7 | R5.2 41.28,25.52 41.9,24.9 R7.2 R8.2 41.9,21.73 42.63,21 IC8.14 | IC9.14 53.74,22.34 v53.72,22.35 52.46,23.61 R18.2 49.67,23.61 R21.2 45.22,23.63 43.58,21.99 IC8.14 | IC8.14 IC8.13 IC8.12 R17.2
  Bottom 0.203: v8.26,21.08 v10.79,21.08 v16.51,21.08
  Bottom 0.254: v16.51,21.08 v24.13,21.08 25.15,20.07 v29.46,20.07 33.02,16.51 v34.92,16.51 38.73,12.7 v49.53,12.7 | v70.48,19.68 v67.94,19.68 v62.23,19.68 56.39,19.68 v53.72,22.35 | v35.94,38.86 v30.73,38.86 | v20.32,52.58 20.95,52.58 24.13,49.4 v24.13,43.81
VCC5V  (via drill 0.35)
  Top 0.254: IC3.7 11.22,17.48 v10.79,17.91 | IC3.18 16.72,17.7 v16.51,17.91 | v24.13,17.91 24.55,17.48 IC4.7 | v29.84,17.91 30.05,17.7 IC4.18 | v61.59,17.14 62.02,16.72 62.02,16.51 IC5.7 | v67.31,17.14 67.52,16.93 IC5.18 | C4.2 74.76,19.68 v73.03,19.68 | C4.2 74.8,17.91 v74.93,17.78 | C4.2 74.87,19.66 IC7.3 | R1.1 57.4,13.59 v57.02,13.21
  Bottom 0.254: EDGE1.A2 5.08,6.99 3.81,8.26 3.81,14.61 7.11,17.91 v10.79,17.91 v16.51,17.91 v24.13,17.91 v29.84,17.91 35.69,12.06 40.01,12.06 41.48,10.59 54.41,10.59 v57.02,13.21 60.96,17.14 v61.59,17.14 62.23,17.14 v67.31,17.14 71.75,17.14 73.03,18.41 v73.03,19.68 | EDGE1.A31 JP2.1 74.93,13.34 v74.93,17.78

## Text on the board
tPlace: + | + | Prototype Game Development Cartridge / for Sega Mega Drive / Genesis / Designed by Mathew Carr / 2020-02-14 Rev. 1 | + | +
bPlace: Prototype Game Development Cartridge / for Sega Mega Drive / Genesis / Designed by Mathew Carr / 2020-02-14 Rev. 1
tNames: 1 | 1 / 2 | 5V GND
